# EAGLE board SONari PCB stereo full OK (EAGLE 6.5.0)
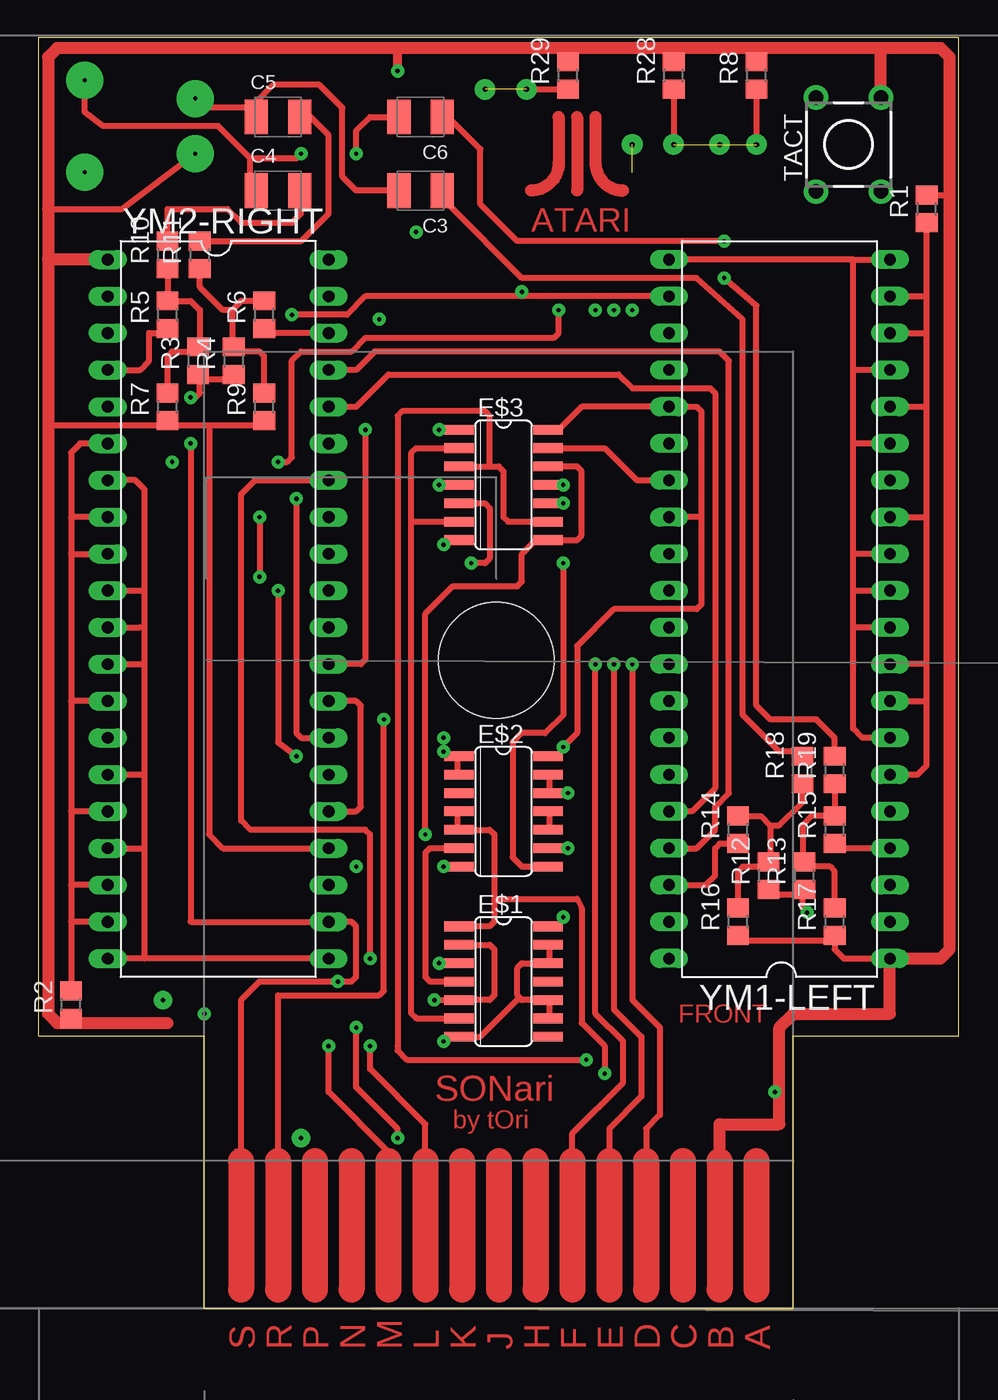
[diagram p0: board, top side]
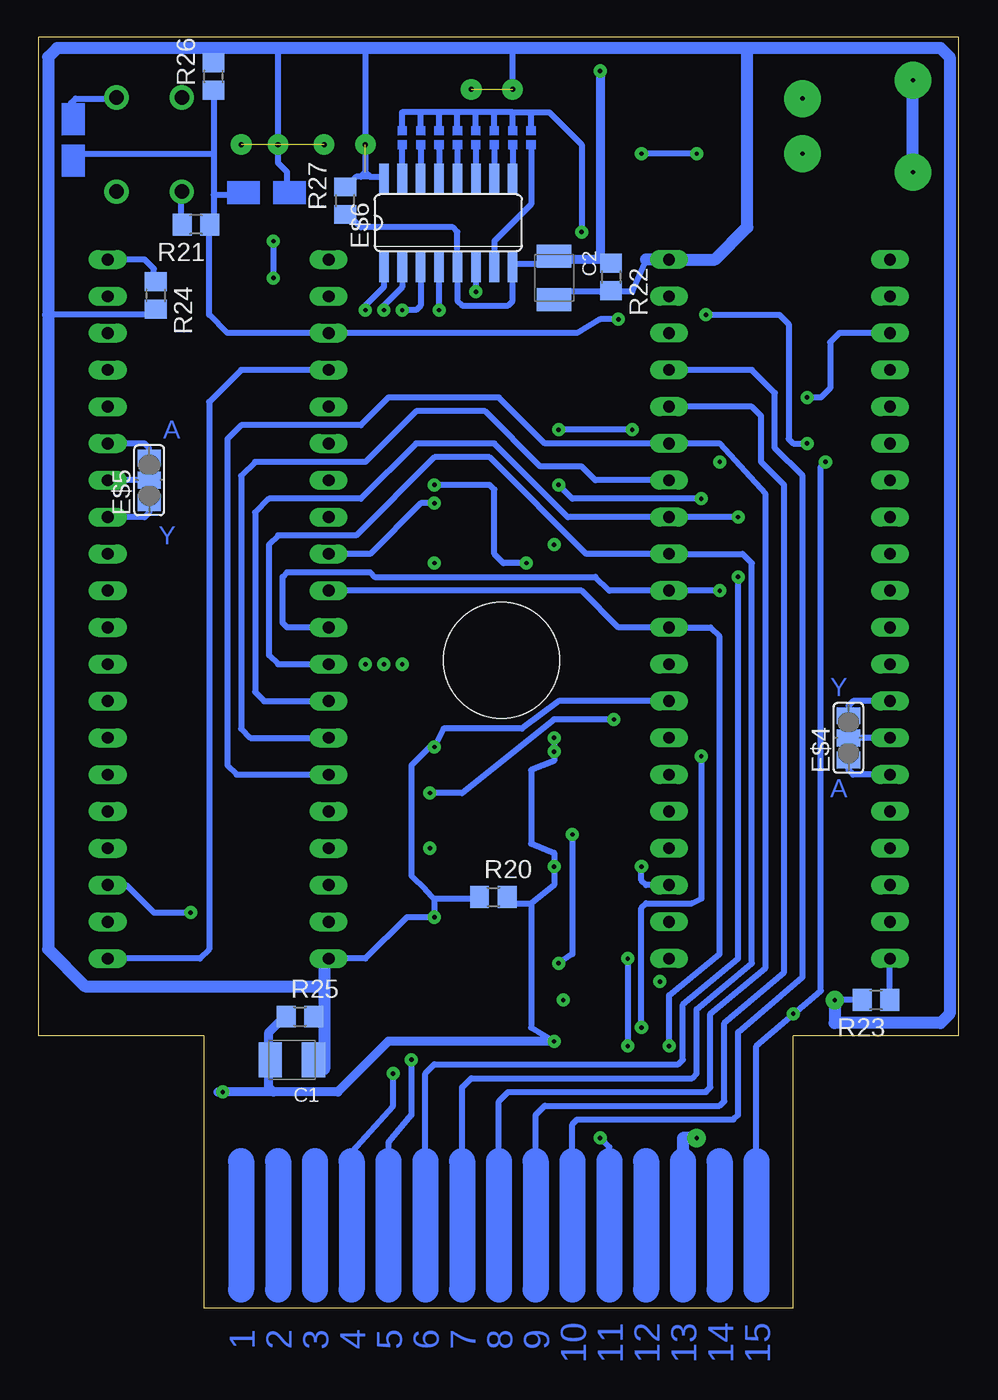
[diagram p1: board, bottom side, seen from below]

Size 63.5 x 87.73 mm. Coordinates in mm from the lower left corner, seen from the top.
Outline: 11.43,0 52.07,0 52.07,18.78 63.5,18.78 63.5,87.73 0,87.73 0,18.78 11.43,18.78 11.43,0
Copper layers (1*16): Top 0.035mm / dielectric 1.5mm / Bottom 0.035mm
Design rules "default": minimum track width 10mil, minimum drill 24mil, track to track 8mil, track to pad 8mil, pad to pad 8mil, via to via 8mil, smd to smd 8mil, copper to edge 40mil, drill to drill 8mil, minimum pad ring 10mil, minimum via ring 8mil, stop-mask expansion 4mil, vias tented up to drill 0mil, thermal gap 10mil
Holes 8 mm at 31.57,44.72

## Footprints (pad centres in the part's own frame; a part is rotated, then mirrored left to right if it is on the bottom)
SMC_B = smd 1.6 x 2.4: + -1.5,0; - 1.5,0
SO14 = smd 0.66 x 2.032: 1 -3.81,-3.073; 2 -2.54,-3.073; 3 -1.27,-3.073; 4 0,-3.073; 5 1.27,-3.073; 6 2.54,-3.073; 7 3.81,-3.073; 8 3.81,3.073; 9 2.54,3.073; 10 1.27,3.073; 11 0,3.073; 12 -1.27,3.073; 13 -2.54,3.073; 14 -3.81,3.073
SJ_2 = smd 1.168 x 1.6: 1 -1.524,0; 2 0,0; 3 1.524,0
SO16 = smd 0.66 x 2.032: 1 -4.445,-3.073; 2 -3.175,-3.073; 3 -1.905,-3.073; 4 -0.635,-3.073; 5 0.635,-3.073; 6 1.905,-3.073; 7 3.175,-3.073; 8 4.445,-3.073; 9 4.445,3.073; 10 3.175,3.073; 11 1.905,3.073; 12 0.635,3.073; 13 -0.635,3.073; 14 -1.905,3.073; 15 -3.175,3.073; 16 -4.445,3.073
R0805 = smd 1.3 x 1.5: 1 -0.95,0; 2 0.95,0
TL1105 = drill 1 pad 1.676: 1 -2.25,3.25; 2 2.25,3.25; 3 -2.25,-3.25; 4 2.25,-3.25
DIL40 = drill 0.813 long: 1 -24.13,-7.62; 2 -21.59,-7.62; 3 -19.05,-7.62; 4 -16.51,-7.62; 5 -13.97,-7.62; 6 -11.43,-7.62; 7 -8.89,-7.62; 8 -6.35,-7.62; 9 -3.81,-7.62; 10 -1.27,-7.62; 11 1.27,-7.62; 12 3.81,-7.62; 13 6.35,-7.62; 14 8.89,-7.62; 15 11.43,-7.62; 16 13.97,-7.62; 17 16.51,-7.62; 18 19.05,-7.62; 19 21.59,-7.62; 20 24.13,-7.62; 21 24.13,7.62; 22 21.59,7.62; 23 19.05,7.62; 24 16.51,7.62; 25 13.97,7.62; 26 11.43,7.62; 27 8.89,7.62; 28 6.35,7.62; 29 3.81,7.62; 30 1.27,7.62; 31 -1.27,7.62; 32 -3.81,7.62; 33 -6.35,7.62; 34 -8.89,7.62; 35 -11.43,7.62; 36 -13.97,7.62; 37 -16.51,7.62; 38 -19.05,7.62; 39 -21.59,7.62; 40 -24.13,7.62

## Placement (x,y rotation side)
C1  10uF  [SMC_B]  46.04,17.14 180 bottom
C2  10uF  [SMC_B]  27.94,71.12 270 bottom
C3  10uF  [SMC_B]  26.35,77.15 180 top
C4  10uF  [SMC_B]  16.51,77.15 0 top
C5  10uF  [SMC_B]  16.51,82.23 0 top
C6  10uF  [SMC_B]  26.35,82.23 180 top
E$1  [SO14]  32.07,22.54 270 top
E$2  [SO14]  32.07,34.29 270 top
E$3  [SO14]  32.07,56.83 270 top
E$4  [SJ_2]  7.62,39.37 90 bottom
E$5  [SJ_2]  55.88,57.15 90 bottom
E$6  [SO16]  35.24,74.93 0 bottom
R1  2k2  [R0805]  61.28,75.88 90 top
R2  2k2  [R0805]  2.22,20.95 90 top
R3  2k2  [R0805]  10.99,65.41 90 top
R4  2k2  [R0805]  13.46,65.41 90 top
R5  1k  [R0805]  8.89,68.58 90 top
R6  1k  [R0805]  15.56,68.58 90 top
R7  1k  [R0805]  8.89,62.23 90 top
R8  330R  [R0805]  49.53,85.09 90 top
R9  1k  [R0805]  15.56,62.23 90 top
R10  2k2  [R0805]  8.89,72.71 90 top
R11  2k2  [R0805]  11.11,72.71 90 top
R12  2k2  [R0805]  50.36,29.84 90 top
R13  2k2  [R0805]  52.83,29.84 90 top
R14  1k  [R0805]  48.26,33.02 90 top
R15  1k  [R0805]  54.93,33.02 90 top
R16  1k  [R0805]  48.26,26.67 90 top
R17  1k  [R0805]  54.93,26.67 90 top
R18  2k2  [R0805]  52.71,37.15 90 top
R19  2k2  [R0805]  54.93,37.15 90 top
R20  0.1uF  [R0805]  32.13,28.38 0 bottom
R21  330R  [R0805]  52.64,74.8 180 bottom
R22  0.1uF  [R0805]  24,71.18 270 bottom
R23  2k2  [R0805]  5.71,21.27 180 bottom
R24  2k2  [R0805]  55.44,69.91 270 bottom
R25  0.1uF  [R0805]  45.47,20.13 0 bottom
R26  5k6  [R0805]  51.44,85.03 90 bottom
R27  0.1uF  [R0805]  42.35,76.45 90 bottom
R28  330R  [R0805]  43.81,85.09 90 top
R29  330R  [R0805]  36.51,85.09 90 top
TACT  RESET  [TL1105]  55.88,80.33 0 top
YM1-LEFT  [DIL40]  51.12,48.26 90 top
YM2-RIGHT  [DIL40]  12.38,48.26 270 top

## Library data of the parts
C1-C6 R1-R29 = rcl
E$1-E$3 E$6 YM1-LEFT YM2-RIGHT = 74xx-us
E$4 E$5 = jumper
TACT = switch

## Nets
S$1: YM1-LEFT.38
S$2: YM2-RIGHT.34
S$7: YM2-RIGHT.6 YM2-RIGHT.8 YM2-RIGHT.9 YM2-RIGHT.13 YM2-RIGHT.16 YM2-RIGHT.18 YM2-RIGHT.19
S$8: YM2-RIGHT.7 YM2-RIGHT.10 YM2-RIGHT.12 YM2-RIGHT.15 YM2-RIGHT.17 YM2-RIGHT.20 YM2-RIGHT.21
S$11: YM2-RIGHT.11
S$15: YM2-RIGHT.4
S$22: YM2-RIGHT.38
S$26: YM1-LEFT.3
S$30: YM2-RIGHT.3
S$34: E$4.2 YM2-RIGHT.14
S$35: E$5.2 YM1-LEFT.14
S$39: YM1-LEFT.8 YM1-LEFT.9 YM1-LEFT.13 YM1-LEFT.16 YM1-LEFT.18 YM1-LEFT.19
S$75: YM1-LEFT.7 YM1-LEFT.10 YM1-LEFT.11 YM1-LEFT.12 YM1-LEFT.15 YM1-LEFT.17 YM1-LEFT.20 YM1-LEFT.21
S$76: YM1-LEFT.33 YM2-RIGHT.33
S$81: YM2-RIGHT.25 YM2-RIGHT.28
S$89: YM1-LEFT.25 YM2-RIGHT.40
S$90: YM1-LEFT.29
S$91: YM1-LEFT.27
S$93: YM2-RIGHT.29
S$94: YM1-LEFT.32 YM2-RIGHT.32
S$95: YM2-RIGHT.27
S$96: YM1-LEFT.37 YM2-RIGHT.37
S$98: YM1-LEFT.31 YM2-RIGHT.31
S$99: YM1-LEFT.30 YM2-RIGHT.30
S$100: YM1-LEFT.36 YM2-RIGHT.36
S$101: YM1-LEFT.35 YM2-RIGHT.35
S$104: YM1-LEFT.22 YM2-RIGHT.22
S$110: YM1-LEFT.1 YM1-LEFT.24 YM2-RIGHT.1
S$112: YM2-RIGHT.24
S$134: YM2-RIGHT.23
S$135: YM1-LEFT.23

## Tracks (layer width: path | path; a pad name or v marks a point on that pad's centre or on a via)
S$1
  Top 0.406: YM1-LEFT.38 46.04,29.21 46.67,29.84 46.67,31.75 46.99,32.07 48.58,32.07
S$2  (via drill 0.3 pad 0.9)
  Top 0.406: 26.67,10.16 26.67,12.7 22.86,16.51 v22.86,18.1 | v22.86,24.13 22.86,32.7 22.54,33.02 14.61,33.02 13.97,33.66 13.97,56.2 14.92,57.15 YM2-RIGHT.34
  Top 1.778: 26.67,10.16 26.67,1.27
  Bottom 0.406: v22.86,24.13 v22.86,18.1 | 43.18,39.37 48.9,39.37 49.53,40 49.53,57.47 48.58,58.42 40.96,58.42 37.47,61.91 32.7,61.91 28.89,58.1 26.04,58.1 25.08,57.15 YM2-RIGHT.34
S$3  (via drill 0.3 pad 0.9)
  Top 0.406: 24.77,18.1 24.77,17.78 25.4,17.14 v37.78,17.14
  Bottom 0.406: 39.37,10.8 39.37,11.43 37.78,13.34 v37.78,17.14
S$4
  Top 0.406: 61.28,76.83 62.55,76.83
S$6
  Top 0.406: 29.53,25.08 31.12,25.08 31.43,24.77 31.43,21.59 31.12,21.27 29.53,21.27
S$7
  Top 0.406: YM2-RIGHT.6 2.86,59.69 2.22,59.05 2.22,54.61 | 2.22,54.61 2.22,52.07 | 2.22,52.07 2.22,41.91 | 2.22,41.91 2.22,34.29 | 2.22,34.29 2.22,29.21 | 2.22,29.21 2.22,26.67 | 2.22,26.67 2.22,22.54 | YM2-RIGHT.8 2.22,54.61 | 2.22,52.07 YM2-RIGHT.9 | YM2-RIGHT.13 2.22,41.91 | YM2-RIGHT.19 2.22,26.67 | YM2-RIGHT.18 2.22,29.21 | YM2-RIGHT.16 2.22,34.29
  Bottom 0.406: YM2-RIGHT.13 7.3,41.91 7.62,41.59 7.62,40.64
S$8
  Top 0.406: YM2-RIGHT.21 7.3,24.13 | 7.3,24.13 YM2-RIGHT.20 | 7.3,24.13 7.3,31.75 | 7.3,31.75 7.3,36.83 | 7.3,36.83 7.3,44.45 | 7.3,44.45 7.3,49.53 | 7.3,49.53 7.3,56.52 6.67,57.15 YM2-RIGHT.7 | YM2-RIGHT.10 7.3,49.53 | YM2-RIGHT.12 7.3,44.45 | YM2-RIGHT.15 7.3,36.83 | YM2-RIGHT.17 7.3,31.75
  Bottom 0.406: YM2-RIGHT.15 7.3,36.83 7.62,37.15 7.62,37.47 | 4.76,21.27 YM2-RIGHT.20
S$9  (via drill 0.3 pad 2.54)
  Top 0.406: 14.61,82.87 11.43,82.87 v10.8,83.5
S$10
  Top 0.406: 28.26,31.75 26.99,31.75 26.67,31.43 26.67,22.86 26.99,22.54 28.58,22.54
S$11
  Top 0.406: YM2-RIGHT.11 6.98,46.99
S$12
  Top 0.813: 37.15,82.23 37.15,77.15
S$13
  Top 0.406: 13.02,64.77 13.34,64.45
S$14
  Bottom 1.778: 34.29,10.16 34.29,1.27
S$15
  Top 0.406: YM2-RIGHT.4 6.98,64.77 7.62,65.41 7.62,67.31 8.57,67.31
S$16
  Bottom 1.778: 31.75,10.16 31.75,1.27
S$17
  Top 1.778: 16.51,10.16 16.51,1.27
S$18
  Top 0.406: 8.89,69.53 10.48,69.53 11.11,68.9 11.11,66.67
S$19
  Bottom 1.778: 29.21,10.16 29.21,1.27
S$20
  Top 0.406: 15.56,69.53 13.97,69.53 13.34,68.9 | 13.34,68.9 13.34,66.67 | 13.34,68.9 12.7,68.9 11.11,70.48 11.11,71.44
S$21
  Bottom 1.778: 26.67,10.16 26.67,1.27
S$22
  Top 0.406: YM2-RIGHT.38 15.88,67.31
S$23
  Top 0.406: 0.95,60.96 15.56,60.96
S$24
  Top 0.406: 8.89,63.82 8.89,65.72 9.21,66.04 10.48,66.04
S$25
  Top 0.406: 15.56,63.5 15.56,65.72 15.24,66.04 13.65,66.04
S$26  (via drill 0.3 pad 0.9)
  Top 0.406: v53.02,27.3 52.71,27.62 52.71,28.58
  Bottom 0.406: YM1-LEFT.3 57.47,29.21 55.56,27.3 v53.02,27.3
S$27
  Top 0.406: 8.89,73.98 8.89,75.88 13.02,75.88 13.97,74.93 17.46,74.93 18.1,75.56 18.1,76.52
S$28
  Top 1.778: 24.13,10.16 24.13,1.27
S$29
  Bottom 1.778: 24.13,10.16 24.13,1.27
S$30  (via drill 0.3 pad 0.9)
  Top 0.406: v10.48,62.86 10.8,62.86 11.11,63.18 11.11,64.14 13.02,64.14
  Bottom 0.406: YM2-RIGHT.3 8.25,67.31 8.89,66.67 8.89,63.5 9.52,62.86 v10.48,62.86
S$31
  Bottom 1.778: 13.97,10.16 13.97,1.27
S$32
  Top 1.778: 13.97,10.16 13.97,1.27
S$33
  Bottom 1.778: 16.51,10.16 16.51,1.27
S$34
  Bottom 0.406: YM2-RIGHT.14 E$4.2
S$35
  Bottom 0.406: E$5.2 YM1-LEFT.14
S$36
  Top 1.778: 19.05,10.16 19.05,1.27
S$37
  Bottom 1.778: 21.59,10.16 21.59,1.27
S$38
  Top 1.778: 21.59,10.16 21.59,1.27
S$39
  Top 0.406: 58.74,36.83 60.64,36.83 61.28,37.47 61.28,41.91 | 61.28,41.91 61.28,44.45 | 61.28,44.45 61.28,54.61 | 61.28,54.61 61.28,62.23 | 61.28,62.23 61.28,67.31 | 61.28,67.31 61.28,69.85 | 61.28,69.85 61.28,74.61 | 61.28,44.45 YM1-LEFT.9 | YM1-LEFT.13 61.28,54.61 | YM1-LEFT.19 61.28,69.85 | YM1-LEFT.18 61.28,67.31 | YM1-LEFT.16 61.28,62.23 | YM1-LEFT.8 61.28,41.91
  Bottom 0.406: 55.88,55.25 55.88,54.93 56.2,54.61 YM1-LEFT.13
S$40  (via drill 0.3 pad 0.9)
  other vias: 50.8,14.92
S$41
  Top 0.406: 8.89,71.44 8.89,70.17
S$42  (via drill 0.3 pad 0.9)
  Top 0.406: v24.77,11.75 24.77,12.38 21.91,15.24 21.91,19.37
  Bottom 0.406: 24.13,10.48 24.13,11.11 v24.77,11.75
S$43
  Top 0.406: 28.89,33.97 28.89,33.34
S$44
  Top 1.778: 29.21,10.16 29.21,1.27
S$45
  Top 0.406: 52.39,29.21 52.71,28.89
S$46
  Top 1.778: 31.75,10.16 31.75,1.27
S$47
  Top 0.406: 48.26,33.97 49.85,33.97 50.48,33.34 | 50.48,33.34 50.48,31.11 | 50.48,33.34 51.12,33.34 52.71,34.92 52.71,35.88
S$48
  Top 1.778: 34.29,10.16 34.29,1.27
S$49
  Top 0.406: 54.93,33.97 53.34,33.97 52.71,33.34 52.71,31.11
S$50  (via drill 0.3 pad 0.9)
  Top 0.406: 36.83,10.16 36.83,12.06 40.32,15.56 40.32,18.41 38.42,20.32 v38.42,44.45
  Top 1.778: 36.83,10.16 36.83,1.27
S$51
  Bottom 1.778: 39.37,10.16 39.37,1.27
S$52
  Top 1.778: 39.37,10.16 39.37,1.27
S$53
  Bottom 1.778: 41.91,10.16 41.91,1.27
S$54
  Top 1.778: 41.91,10.16 41.91,1.27
S$55
  Bottom 1.778: 44.45,10.16 44.45,1.27
S$56
  Top 1.778: 44.45,10.16 44.45,1.27
S$57
  Bottom 1.778: 46.99,10.16 46.99,1.27
S$58
  Top 0.406: 59.37,31.75 55.24,31.75
S$59
  Bottom 1.778: 49.53,10.16 49.53,1.27
S$60
  Top 1.778: 49.53,10.16 49.53,1.27
S$61
  Bottom 0.406: 24.77,70.17 27.3,70.17
S$62  (via drill 0.3 pad 0.9)
  Top 0.406: 29.53,33.02 31.12,33.02 31.43,32.7 31.43,28.26 | 31.43,28.26 31.43,26.67 31.12,26.35 29.53,26.35 | 31.43,28.26 37.15,28.26 37.47,27.62 37.47,19.69 39.05,18.1 v39.05,16.19
  Bottom 0.406: 41.91,10.8 39.05,13.97 v39.05,16.19
S$63
  Top 0.406: 48.26,28.26 48.26,30.16 48.58,30.48 49.85,30.48
S$64
  Top 0.406: 54.93,27.94 54.93,30.16 54.61,30.48 53.02,30.48
S$65
  Top 0.406: 50.48,28.58 52.39,28.58
S$66  (via drill 0.3 pad 0.9)
  Bottom 0.406: v35.88,68.9 35.88,71.12 | 33.34,70.8 v33.34,70.17
S$67
  Top 0.406: 54.93,35.88 54.93,34.29
S$68
  Top 0.406: 28.89,38.1 28.89,36.83
S$69
  Top 0.406: 35.24,34.29 35.24,33.02
S$70  (via drill 0.3 pad 1.27)
  Bottom 0.813: v18.1,11.75 19.05,11.75 19.05,10.16
  Bottom 1.778: 19.05,10.16 19.05,1.27
S$71
  Top 0.406: 35.24,36.83 35.24,35.56
S$72
  Top 0.406: 35.88,53.02 37.15,53.02 37.47,53.34 37.47,57.78 37.15,58.1 35.88,58.1
S$73
  Top 0.406: 29.84,58.1 31.12,58.1 | 31.12,58.1 31.75,58.1 32.07,57.78 32.07,54.61 32.38,54.29 34.29,54.29 | 31.12,58.1 31.12,61.59 30.8,61.91 25.08,61.91 24.77,61.59 24.77,18.1
S$74
  Top 0.406: 23.81,40.64 23.81,21.91 23.49,21.59 16.51,21.59 16.51,10.8
S$75
  Top 0.406: YM1-LEFT.7 56.83,39.37 56.2,40 56.2,46.99 | 56.2,46.99 56.2,49.53 | 56.2,49.53 56.2,52.07 | 56.2,52.07 56.2,59.69 | 56.2,59.69 56.2,64.77 | 56.2,64.77 56.2,72.39 | 56.2,72.39 YM1-LEFT.20 | 56.2,72.39 YM1-LEFT.21 | YM1-LEFT.10 56.2,46.99 | 56.2,49.53 YM1-LEFT.11 | YM1-LEFT.12 56.2,52.07 | YM1-LEFT.15 56.2,59.69 | YM1-LEFT.17 56.2,64.77
  Bottom 0.406: 55.56,71.12 55.56,71.75 56.2,72.39 YM1-LEFT.20 | 55.88,59.05 55.88,59.37 56.2,59.69 YM1-LEFT.15
S$76  (via drill 0.3 pad 0.9)
  Top 0.406: v15.24,54.61 v15.24,50.48
  Bottom 0.406: YM1-LEFT.33 47.94,41.91 48.58,42.55 48.58,54.93 47.62,55.88 41.27,55.88 37.47,59.69 32.07,59.69 26.99,54.61 YM2-RIGHT.33 v15.24,54.61 | 36.83,10.16 36.83,16.19 36.2,16.83 19.37,16.83 19.05,17.14 19.05,20.95 15.24,24.13 v15.24,50.48
  Bottom 1.778: 36.83,10.16 36.83,1.27
S$77
  Top 0.406: 35.24,21.27 35.24,20.32
S$78
  Top 0.406: 35.24,25.08 35.24,23.81
S$79
  Top 0.406: 34.29,21.27 33.34,21.27 33.02,21.59 33.02,23.5 33.34,23.81 34.92,23.81
S$80
  Top 0.406: 29.53,18.73 30.48,18.73 33.02,21.27
S$81
  Top 0.406: YM2-RIGHT.25 21.91,34.29 22.23,34.61 22.23,41.59 21.91,41.91 YM2-RIGHT.28
S$82  (via drill 0.3 pad 0.9)
  Top 0.406: v26.67,32.7 26.67,47.94 28.58,49.85 33.02,49.85 33.34,50.17 33.34,52.07 34.29,53.02
  Bottom 0.406: v26.67,32.7 26.67,24.45 v27.62,23.81
S$83  (via drill 0.3 pad 0.9)
  Top 0.406: 29.84,55.56 30.8,55.56 31.12,55.25 31.12,51.75 30.8,51.44 v29.84,51.44 | v36.2,51.44 36.2,40.96 34.92,39.69 33.34,39.69 32.7,39.05 32.7,31.11 33.34,30.48 34.29,30.48
  Bottom 0.406: v29.84,51.44 31.43,51.44 32.07,52.07 32.07,56.52 32.38,56.83 v36.2,56.83
S$84  (via drill 0.3 pad 0.9)
  other vias: 27.94,52.7
S$85  (via drill 0.3 pad 0.9)
  Top 0.406: v39.69,44.45 39.69,20.64 41.59,18.73 41.59,14.6 39.37,12.38 39.37,10.48
S$87
  Top 0.406: 25.72,54.29 25.72,20.32 26.04,20 28.26,20 | 25.72,54.29 28.26,54.29 | 25.72,54.29 25.72,59.05 26.04,59.37 28.26,59.37
S$88
  Bottom 0.406: 28.58,72.07 30.8,72.07
S$89  (via drill 0.3 pad 0.9, 0.3 pad 1.27, 0.35 pad 1.42)  (2 unrouted)
  Top 0.406: 45.72,54.61 45.72,61.91 45.4,62.23 YM1-LEFT.25 37.47,62.23 35.88,60.64 | 45.72,54.61 43.18,54.61 | 45.72,54.61 45.72,48.58 45.4,48.26 39.69,48.26 37.15,45.72 37.15,39.69 v36.2,38.73 | v33.66,84.14 36.51,84.14 | 35.88,35.56 v36.51,35.56
  Bottom 0.406: 46.35,77.47 46.35,78.42 46.99,79.06 v46.99,80.33 46.99,87 | 20.32,41.91 27.62,41.91 30.16,40 35.56,40 v36.2,38.73 36.51,38.73 37.78,37.47 37.78,29.84 36.83,28.89 36.2,28.26 | 36.2,28.26 v36.2,26.99 38.1,26.99 40.96,24.13 43.81,24.13 | 33.66,28.26 36.2,28.26 | 21.59,72.39 22.54,70.17 24.77,70.17 | 6.98,21.27 v8.57,21.27 | 55.56,68.58 62.87,68.58 | 40.96,87 40.96,78.42 | 40.96,78.42 40.64,78.11 | 40.64,78.11 39.69,78.11 | 51.44,87 51.44,86.36 | 40.64,78.11 41.27,78.11 | 41.27,78.11 41.59,78.11 42.23,77.47 | 40.96,78.42 41.27,78.11 | v30.8,84.14 30.8,87
  Bottom 0.813: 14.61,87 1.27,87 0.63,86.36 0.63,20.32 1.27,19.69 8.57,19.69 v8.57,21.27 | 14.61,87 30.8,87 40.96,87 46.99,87 51.44,87 62.23,87 62.87,86.36 62.87,68.58 62.87,24.77 60.32,22.23 43.81,22.23 | 21.59,72.39 YM2-RIGHT.40 16.83,72.39 14.61,74.61 14.61,87 | 43.81,24.13 43.81,22.23 | 43.81,22.23 43.81,16.51
  other vias: 40.96,80.33
S$90  (via drill 0.3 pad 0.9)
  Bottom 0.406: v36.2,55.56 37.15,55.56 40.64,52.07 YM1-LEFT.29
S$91
  Top 0.406: 35.88,59.37 39.05,59.37 41.27,57.15 YM1-LEFT.27
S$92  (via drill 0.3 pad 0.9)
  Bottom 0.406: 29.53,27.94 27.94,29.21 v27.94,30.48 27.94,31.43 29.53,32.07 29.53,37.15 27.94,37.78 v27.94,38.42 v27.94,39.37 | 29.53,27.94 29.53,19.37 v27.94,18.41 | 30.8,27.94 29.53,27.94 | v23.81,40.64 27.94,40.64 34.29,35.56 36.51,35.56
  Bottom 0.61: v27.94,18.41 39.37,18.41 42.86,14.92 47.31,14.92 | 47.31,14.92 47.62,15.24 47.62,19.05 46.67,20 | 47.31,14.92 51.12,14.92
S$93  (via drill 0.3 pad 0.9)
  Top 0.406: v22.54,60.64 22.54,44.77 22.23,44.45 YM2-RIGHT.29
  Bottom 0.406: v22.54,60.64 v27.62,60.64
S$94
  Bottom 0.406: YM1-LEFT.32 46.99,44.45 47.62,45.08 47.62,52.7 46.99,53.34 41.59,53.34 36.2,58.74 32.38,58.74 25.72,52.07 YM2-RIGHT.32 14.92,52.07 14.29,51.44 14.29,23.81 18.1,20.64 18.1,16.19 18.41,15.88 33.66,15.88 34.29,15.24 34.29,10.48
S$95  (via drill 0.3 pad 0.9)
  Top 0.406: v17.78,55.88 17.78,39.69 18.1,39.37 YM2-RIGHT.27
  Bottom 0.406: v17.78,55.88 26.67,55.88 v27.62,56.83
S$96
  Top 0.406: YM1-LEFT.37 45.4,31.75 46.67,33.02 46.67,34.61 47.62,35.56 47.62,65.41 46.99,66.04 23.18,66.04 21.91,64.77 YM2-RIGHT.37
S$97
  Bottom 0.406: 26.67,10.48 26.67,12.7 26.35,13.02 15.56,13.02 15.24,13.34 15.24,19.05 10.8,22.86 10.8,57.47 12.7,59.37 12.7,63.18 14.29,64.77 19.68,64.77 20,65.09
S$98  (via drill 0.3 pad 0.9)
  Top 0.406: v16.51,49.53 16.51,39.05 v17.78,38.1
  Bottom 0.406: YM1-LEFT.31 46.35,46.99 46.67,47.31 46.67,50.48 46.35,50.8 40.64,50.8 40.32,50.48 25.08,50.48 24.13,49.53 YM2-RIGHT.31 v16.51,49.53 | v21.91,19.37 21.91,27.62 21.59,27.94 18.41,27.94 17.78,28.26 v17.78,38.1
  other vias: 20.64,22.54 36.51,31.75
S$99  (via drill 0.3 pad 0.9)
  Top 0.406: 24.13,10.48 24.13,10.8 20,14.92 v20,18.1
  Bottom 0.406: YM1-LEFT.30 26.04,49.53 23.49,46.99 YM2-RIGHT.30 17.14,46.99 16.51,46.36 16.51,24.45 20,21.59 v20,18.1
S$100
  Top 0.406: YM2-RIGHT.36 21.91,62.23 24.13,64.45 40.01,64.45 40.96,63.5 46.35,63.5 46.67,63.18 46.67,35.88 45.09,34.29 YM1-LEFT.36
  Bottom 0.406: 29.21,10.48 29.21,13.34 28.58,13.97 16.51,13.97 16.19,14.29 16.19,19.69 12.07,23.18 12.07,56.83 13.65,58.42 13.65,61.59 14.29,62.23 YM2-RIGHT.36
S$101
  Bottom 0.406: 31.75,10.48 31.75,14.29 31.12,14.92 17.46,14.92 17.14,15.24 17.14,20.32 13.34,23.5 13.34,56.2 16.51,59.69 YM2-RIGHT.35 28.58,59.69 31.75,62.86 39.37,62.86 41.27,60.96 49.53,60.96 50.48,60.01 50.48,37.47 49.85,36.83 YM1-LEFT.35
S$102
  Top 0.406: 11.11,73.66 18.1,73.66 20,75.56 20,80.96 18.41,82.55
S$103  (via drill 0.3 pad 0.9)
  Top 0.406: v40.96,44.45 40.96,21.27 42.86,19.37 42.86,13.34 41.91,12.38 41.91,10.48
S$104  (via drill 0.3 pad 0.9)
  Top 0.406: 13.97,10.8 13.97,21.27 15.24,22.54 21.59,22.54 21.91,22.86 21.91,26.35 21.59,26.67 YM2-RIGHT.22 10.48,26.67 v10.48,59.69 | YM1-LEFT.22 22.54,69.85 21.27,68.58 v17.46,68.58
  Bottom 0.406: v17.46,68.58 12.38,68.58 11.75,67.94 11.75,60.01 11.43,59.69 v10.48,59.69
S$105
  Top 0.406: 13.65,10.48 13.65,10.8
S$106  (via drill 0.3 pad 0.9)
  Top 0.406: v47.31,73.66 33.02,73.66 30.48,76.2 30.48,80.01 28.26,82.23 | 54.93,38.42 54.93,39.37 53.66,40.64 50.48,40.64 49.53,41.59 49.53,69.22 v47.31,71.12
  Bottom 0.406: v47.31,73.66 v47.31,71.12
S$107
  Top 0.406: 52.71,38.42 51.12,38.42 48.58,40.96 48.58,68.26 45.4,71.12 33.34,71.12 28.26,76.2
S$108  (via drill 0.3 pad 0.9, 0.3 pad 2.54)
  Top 0.406: v3.18,84.77 3.18,82.55 4.45,81.6 12.38,81.6 14.61,79.38 | 14.61,78.11 14.61,79.38 | 14.61,79.38 17.78,79.38 v18.1,79.69 | v21.91,79.69 21.91,81.28 22.86,82.23 25.08,82.23
  Bottom 0.406: v18.1,79.69 v21.91,79.69
  Bottom 0.813: v3.18,78.42 v3.18,84.77
S$109
  Bottom 0.406: 30.8,81.28 30.8,82.55 | 30.8,82.55 32.07,82.55 | 32.07,82.55 33.34,82.55 | 33.34,82.55 34.61,82.55 | 34.61,82.55 35.88,82.55 | 35.88,82.55 37.15,82.55 | 37.15,82.55 38.42,82.55 38.42,81.28 | 37.15,81.28 37.15,82.55 | 35.88,81.28 35.88,82.55 | 34.61,81.28 34.61,82.55 | 33.34,81.28 33.34,82.55 | 32.07,81.28 32.07,82.55 | 30.8,82.55 29.53,82.55 | 29.53,82.55 28.26,82.55 26.04,80.33 26.04,74.3 | 29.53,81.28 29.53,82.55
S$110  (via drill 0.3 pad 0.9, 0.3 pad 2.54)
  Top 0.406: 48.26,25.4 54.93,25.4 54.93,24.77 55.56,24.13 YM1-LEFT.1 | 0.63,75.88 5.71,75.88 v10.8,79.69 | 49.53,87 49.53,86.36
  Top 0.61: v24.77,85.41 24.77,87
  Top 0.813: 46.99,10.16 46.99,12.7 51.12,12.7 51.12,19.37 52.07,20.32 58.74,20.32 YM1-LEFT.1 62.23,24.13 62.87,24.77 62.87,86.36 62.23,87 58.1,87 | 58.1,87 49.53,87 24.77,87 1.27,87 0.63,86.36 0.63,75.88 0.63,72.39 | 0.63,72.39 0.63,20.32 1.27,19.69 8.89,19.69 | 58.1,83.5 58.1,87 | YM2-RIGHT.1 0.63,72.39
  Top 1.778: 46.99,10.16 46.99,1.27
  Bottom 0.406: YM1-LEFT.24 49.53,64.77 51.75,62.55 51.75,24.77 52.39,24.13 YM1-LEFT.1
  Bottom 0.61: v24.77,85.41 24.77,72.39 27.3,72.39
S$111
  Top 0.406: 24.45,77.15 21.91,77.15 20.95,78.11 20.95,82.87 19.37,84.45 16.19,84.45 14.92,83.19
S$112
  Top 0.406: 11.75,60.96 11.75,32.7 12.7,31.75 YM2-RIGHT.24
S$113
  Bottom 0.406: 34.61,71.12 34.61,69.53 34.29,69.22 31.12,69.22 30.8,69.53 30.8,71.44
S$114  (via drill 0.3 pad 0.9)
  Top 0.406: v16.51,58.42 17.14,58.42 17.46,58.74 17.46,65.41 18.1,66.04 21.59,66.04 22.54,66.99 35.56,66.99 35.88,67.31 35.88,68.9
S$115  (via drill 0.3 pad 0.9)
  Bottom 0.406: v9.21,58.42 9.52,58.1 9.52,21.91 13.97,18.1 13.97,10.48
S$116  (via drill 0.3 pad 0.9)
  Bottom 0.406: 37.15,71.12 37.15,69.22 37.47,68.9 v38.42,68.9
S$117  (via drill 0.3 pad 0.9)
  Bottom 0.406: 38.42,71.12 38.42,70.48 39.69,69.22 v39.69,68.9
S$118  (via drill 0.3 pad 0.9)
  Bottom 0.406: 39.69,71.12 39.69,70.48 40.96,69.22 v40.96,68.9
S$120
  Bottom 0.406: 38.42,78.42 38.42,80.01
S$121
  Bottom 0.406: 37.15,80.01 37.15,78.74
S$122
  Bottom 0.406: 35.88,80.01 35.88,78.74
S$123
  Bottom 0.406: 34.61,80.01 34.61,78.74
S$124
  Bottom 0.406: 33.34,80.01 33.34,79.06
S$125
  Bottom 0.406: 32.07,80.01 32.07,79.06
S$126
  Bottom 0.406: 30.8,80.01 30.8,78.74
S$127  (via drill 0.3 pad 0.9)
  other vias: 26.04,74.3
S$128  (via drill 0.3 pad 0.9)
  Top 0.406: v27.3,21.27 28.26,21.27
S$129
  Top 0.813: 38.42,82.23 38.42,79.06 arc90 40.32,77.15
S$130
  Bottom 0.406: 53.66,74.93 53.66,77.15
S$131
  Bottom 0.406: 51.44,83.82 51.44,79.69 | 51.44,79.69 51.44,76.83 | 51.44,76.83 51.44,75.25 | 61.28,79.69 51.44,79.69 | 50.16,76.83 51.44,76.83
S$132
  Bottom 0.406: 61.28,81.6 61.28,83.19 60.96,83.5 58.1,83.5
S$133  (via drill 0.3 pad 0.9)
  other vias: 11.43,20.32
S$134  (via drill 0.3 pad 0.9)
  Bottom 0.406: YM2-RIGHT.23 21.59,29.21 21.91,29.53 v21.91,30.48
S$135  (via drill 0.3 pad 0.9)
  Bottom 0.406: v23.49,68.26 24.77,68.26 26.35,67.31 YM1-LEFT.23 50.48,67.31 51.75,68.58 51.75,74.93
S$136
  Bottom 0.406: 34.61,72.39 34.61,74.3 34.92,74.61 41.27,74.61 41.91,75.25
S$137
  Bottom 0.406: 29.53,80.33 29.53,76.2 32.07,73.66 32.07,72.39
S$138
  Top 0.813: 35.88,82.23 35.88,79.06 arc-90 33.97,77.15
S$150  (via drill 0.35 pad 1.42)  (1 unrouted)
  Top 0.406: 49.53,83.82 v49.53,80.33 | 43.81,83.82 v43.81,80.33
(copper drawn outside any net)
  shapes: Bottom area x28

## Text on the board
Top: ATARI | FRONT | SONari | by tOri | S | R | P | N | M | L | K | J | H | F | E | D | C | B | A
Bottom: A | Y | Y | A | 9 | 8 | 7 | 6 | 5 | 4 | 3 | 2 | 1 | 15 | 14 | 13 | 12 | 11 | 10
tValues: 7402 | 7400 | 7432
bValues: 1uF | D1 | 1uF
